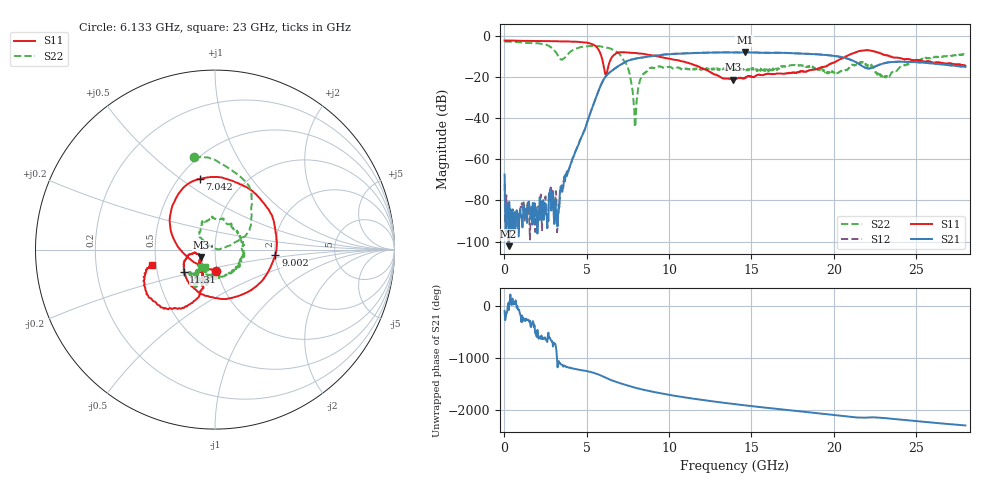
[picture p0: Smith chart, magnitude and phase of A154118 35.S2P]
!  2-Port S-parameters saved by WinCal
! VAR MeasName=S-Parameters (CALIBRATED_DATA) read from VNA (N5230A)
! VAR MeasDate=2015-9-10 14:37:08
! VAR NAME=A154118 35
! VAR FILENAME=A154118 35.S2P
! VAR DATE=2015-9-10 14:37:08
! VAR PHYS_PORTS=1,2
# Hz S DB R 50
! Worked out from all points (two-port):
!   801 points, 10 MHz to 28 GHz, reference 50 ohm
!   highest |S21| = -7.90 dB at 14.6 GHz (marker M1); lowest = -102.2 dB at 254.9 MHz (marker M2)
!   |S21| within 3 dB of the highest: 8.015 GHz to 20.8 GHz (12.79 GHz wide, 88.7 % of centre)
!   lowest |S11| = -21.2 dB at 13.9 GHz (marker M3), VSWR 1.19, Z = 42.7 - j3.56 ohm
!   |S11| at or under -10 dB: 5.894 GHz to 6.56 GHz (666.3 MHz wide, 10.7 % of centre); 9.357 GHz to 20.72 GHz (11.36 GHz wide, 75.5 % of centre); 23.49 GHz to end of sweep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
!   |S22| runs from -44.2 to -2.7 dB; largest |S21 - S12| = 0.0079
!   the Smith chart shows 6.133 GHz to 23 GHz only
!   S11 on the Smith chart (normalised r, x): 6.133 GHz: 0.98, -0.23; 7.042 GHz: 0.63, +0.59; 9.002 GHz: 2.01, -0.14; 11.31 GHz: 0.68, -0.18; 23 GHz: 0.48, -0.09
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1e7  -2.15 179.7  -67.37 -102.3  -71.91 140.9  -2.67 179.8
2.549125e8  -2.18 176.2  -102.23 -85.6  -84.23 107.8  -2.70 173.7
2.459125e9  -2.47 146.9  -83.92 114.2  -79.84 96.8  -4.07 104.9
3.193862e9  -2.51 134.9  -90.96 41.4  -95.43 -89.9  -8.71 25.6
3.753662e9  -2.59 123.8  -67.97 -98.0  -67.91 -99.1  -9.82 -108.6
4.698325e9  -3.01 98.1  -48.87 -159.1  -48.69 -159.0  -5.29 166.5
5.642988e9  -5.78 38.0  -28.12 130.4  -28.06 130.7  -4.94 124.3
6.132812e9  -18.59 -87.6  -19.85 61.6  -19.78 61.6  -5.55 102.9
7.042488e9  -7.90 102.1  -14.01 -46.3  -13.96 -46.7  -9.32 53.3
7.532312e9  -8.06 77.0  -11.91 -94.5  -11.89 -94.6  -16.36 22.8
7.952162e9  -8.23 57.5  -11.00 -132.1  -11.02 -132.2  -44.25 141.1
8.302038e9  -8.58 38.8  -10.52 -160.0  -10.52 -160.2  -20.16 140.0
9.001788e9  -9.44 -5.1  -9.72 152.2  -9.66 152.3  -15.51 111.9
9.351662e9  -10.00 -30.1  -9.41 130.4  -9.33 130.3  -14.79 97.4
1.131096e10  -13.36 -144.1  -8.35 26.5  -8.31 25.6  -15.93 28.8
1.390004e10  -21.19 -151.7  -7.99 -81.7  -7.99 -82.6  -16.10 -72.1
1.4005e10  -21.00 -151.9  -7.97 -85.8  -7.97 -86.4  -16.25 -75.3
1.459979e10  -20.40 -146.3  -7.90 -107.8  -7.88 -108.2  -16.37 -80.0
1.869332e10  -16.41 -118.0  -8.74 112.2  -8.76 111.7  -14.73 -122.9
2.299679e10  -8.87 -166.6  -13.38 11.2  -13.38 10.4  -19.17 -119.4
2.334666e10  -9.69 -169.1  -12.80 0.2  -12.75 -1.0  -19.87 -94.7
2.8e10  -14.56 -165.6  -15.01 -133.4  -15.06 -134.1  -8.61 -112.8
